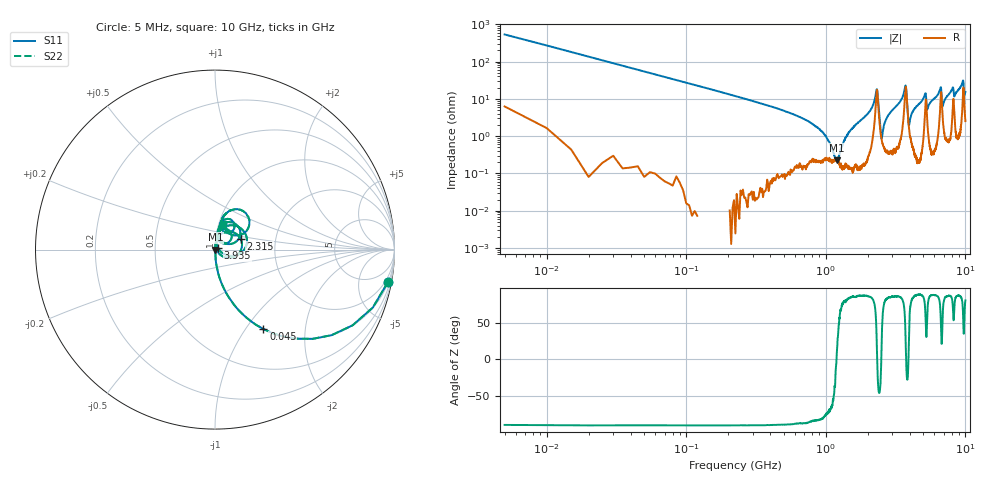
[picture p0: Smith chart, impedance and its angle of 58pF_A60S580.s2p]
! Amotech Co.,Ltd.
! http://www.amotech.co.kr/
! Part Number: A60S580
! These Parameters are Measured in Series Mode Connection
! Operation Temp=25[degC], DC Bias Voltage=0[V]
! Freq. Start=5[MHz] Stop=10[GHz], 2000[Steps]
! Date: Monday, July 13, 2020, 01:43:14
# GHZ S RI R 50.000000
!Freq.(Hz) S11(Real) S11(Imag) S21(Real) S21(Imag) S12(Real) S12(Imag) S22(Real) S22(Imag)
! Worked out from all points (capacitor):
!   2000 points, 5 MHz to 10 GHz, reference 50 ohm
!   read as one part in series: C = 58 pF near 55 MHz
!   lowest |Z| = 223 mohm at 1.2 GHz (marker M1)
!   series resonance near 1.193 GHz, so ESL is about 310 pH
!   S11 on the Smith chart (normalised r, x): 5 MHz: 1, -11; 45 MHz: 1.00, -1.21; 2.315 GHz: 1.32, +0.16; 3.935 GHz: 1.04, +0.02; 10 GHz: 1.05, +0.30
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0.005  0.9644 -0.1794  0.0356 0.1794  0.0356 0.1794  0.9644 -0.1794
0.045  0.2699 -0.4426  0.7301 0.4426  0.7301 0.4426  0.2699 -0.4426
0.17  0.0247 -0.1558  0.9753 0.1558  0.9753 0.1558  0.0247 -0.1558
0.92  0.00222 -0.0141  0.9978 0.0141  0.9978 0.0141  0.00222 -0.0141
1.2  0.00219 0.000399  0.9978 -0.000399  0.9978 -0.000399  0.00219 0.000399
1.675  0.00211 0.0218  0.9979 -0.0218  0.9979 -0.0218  0.00211 0.0218
2.315  0.1426 0.0607  0.8574 -0.0607  0.8574 -0.0607  0.1426 0.0607
2.52  0.00746 0.00476  0.9925 -0.00476  0.9925 -0.00476  0.00746 0.00476
2.775  0.005 0.0336  0.995 -0.0336  0.995 -0.0336  0.005 0.0336
3.34  0.0114 0.0754  0.9886 -0.0754  0.9886 -0.0754  0.0114 0.0754
3.725  0.1711 0.0841  0.8289 -0.0841  0.8289 -0.0841  0.1711 0.0841
3.935  0.0178 0.00821  0.9822 -0.00821  0.9822 -0.00821  0.0178 0.00821
5.005  0.0191 0.1002  0.9809 -0.1002  0.9809 -0.1002  0.0191 0.1002
5.175  0.0791 0.1054  0.9209 -0.1054  0.9209 -0.1054  0.0791 0.1054
5.345  0.0233 0.0464  0.9767 -0.0464  0.9767 -0.0464  0.0233 0.0464
6.67  0.1327 0.1229  0.8673 -0.1229  0.8673 -0.1229  0.1327 0.1229
6.86  0.0375 0.0473  0.9625 -0.0473  0.9625 -0.0473  0.0375 0.0473
8.1  0.0763 0.171  0.9237 -0.171  0.9237 -0.171  0.0763 0.171
8.335  0.0469 0.1019  0.9531 -0.1019  0.9531 -0.1019  0.0469 0.1019
9.585  0.1507 0.2165  0.8493 -0.2165  0.8493 -0.2165  0.1507 0.2165
9.82  0.0791 0.0899  0.9209 -0.0899  0.9209 -0.0899  0.0791 0.0899
10  0.0459 0.1418  0.9541 -0.1418  0.9541 -0.1418  0.0459 0.1418
